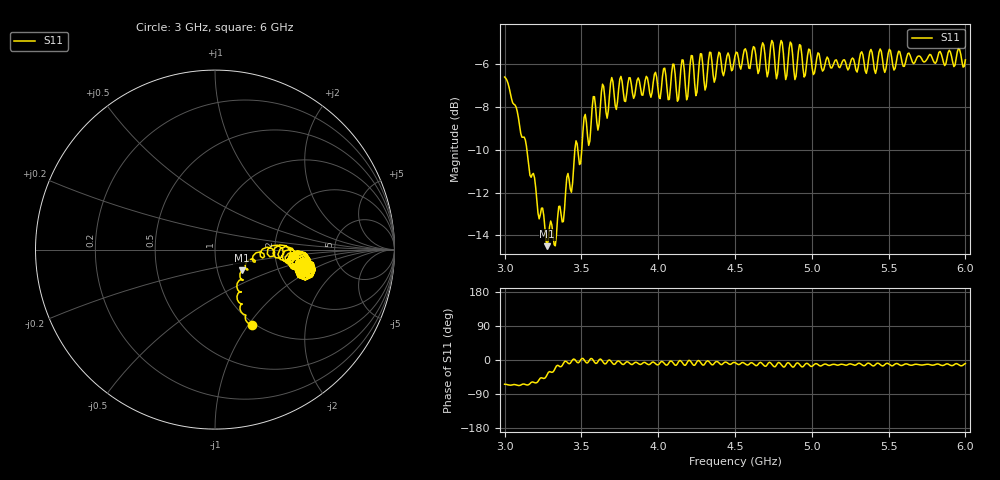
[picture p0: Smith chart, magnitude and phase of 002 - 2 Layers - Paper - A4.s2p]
!  02/07/2025  14:49:10
! Ref Plane: 0.000 mm
# MHZ S MA R  50
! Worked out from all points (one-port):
!   401 points, 3 GHz to 6 GHz, reference 50 ohm
!   lowest |S11| = -14.5 dB at 3.277 GHz (marker M1), VSWR 1.46, Z = 65.3 - j15.7 ohm
!   |S11| at or under -10 dB: 3.145 GHz to 3.457 GHz (312.2 MHz wide, 9.46 % of centre); 3.477 GHz to 3.502 GHz (25.84 MHz wide, 0.741 % of centre)
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3000  0.4679 -64.0
3150  0.3055 -66.0
3277.5  0.1883 -38.1
3375  0.2145 -14.6
3525  0.3827 -3.9
3750  0.4627 -4.6
4095  0.5014 -6.4
4125  0.4107 -9.9
4155  0.5131 -5.8
4185  0.4139 -9.5
4215  0.5252 -5.7
4245  0.4232 -9.6
4275  0.5305 -5.8
4305  0.4362 -9.2
4335  0.5347 -6.1
4500  0.5241 -6.9
4695  0.5287 -16.5
4725  0.5178 -6.0
4755  0.5317 -17.8
4785  0.5144 -6.4
4815  0.5316 -18.5
4845  0.5088 -7.0
4875  0.5287 -18.6
4905  0.5023 -7.5
4935  0.5273 -18.0
5250  0.5035 -10.2
5625  0.5306 -11.2
6000  0.5132 -9.5
